| IBIS file stm32u375_385_wlcsp68-g_smps.ibs
[IBIS ver] 4.2
[File name] stm32u375_385_wlcsp68-g_smps.ibs
[File Rev] 1.2
[Date] 23-06-2025
[Source] Data Created at STMicroelectronics
[Notes]  File originated from ELDO simulations.
[Disclaimer]  This information is for modeling purpose only and is
   not guaranted. The information is subject to change without
   notice.
[Copyright] Copyright 2025 STMicroelectronics Inc.
|   Component stm32u375_385_wlcsp68-g_smps
[Component] stm32u375_385_wlcsp68-g_smps
[Manufacturer] STMicroelectronics
[Package]
| variable   typ   min   max
R_pkg  0  NA  NA
L_pkg  0  NA  NA
C_pkg  0  NA  NA
[Pin]   signal_name   model_name
A1  VDDUSB  power
A3  PG10  io8_ft_100m_hslv
A5  VDDIO2  power
A7  PB7  io8_ft_100m_hslv
A9  VDD  power
B2  VDD  power
B4  PG14  io8_ft_100m_hslv
B6  PB4  io8_ft_100m_hslv
B8  PH3-BOOT0  io8_ft_100m_hslv
C1  PA12  io8usb_ft_phy
C3  PG9  io8_ft_100m_hslv
C5  VSS  gnd
C7  PB6  io8_ft_100m_hslv
C9  VBAT  power
D2  VSS  gnd
D4  PG12  io8_ft_100m_hslv
D6  PB3  io8_ft_100m_hslv
D8  VSS  gnd
E1  PA11  io8usb_ft_phy
E3  PA15  io8_ft_100m
E5  PG13  io8_ft_100m_hslv
E7  PB5  io8_ft_100m_hslv
E9  PC14-OSC32_IN  io_ft_tamp
F2  PA10  io8_ft_100m
F4  PA14  io8_ft_100m
F6  PG15  io8_ft_100m_hslv
F8  PC13  io8_ft_100m_v33
G1  VDDIO2  power
G3  PA9  io8_ft_100m
G5  PG11  io8_ft_100m_hslv
G7  NRST  ioreset_v33
G9  PC15-OSC32_OUT  io_ft_tamp
H2  VSS  gnd
H4  PA13  io8_ft_100m
H6  PA8  io8_ft_100m_hslv
H8  PH1-OSC_OUT  io8_ft_100m
J1  PG6  io8_ft_100m_hslv
J3  PG7  io8_ft_100m_hslv
J5  PG8  io8_ft_100m_hslv
J7  PA0  io8_ft_100m
J9  PH0-OSC_IN  io8_ft_100m
K2  PG4  io8_ft_100m_hslv
K4  PG5  io8_ft_100m_hslv
K6  PA5  io8_ft_100m
K8  VSSA  nc
L1  PG2  io8_ft_100m_hslv
L3  PB15  io8_ft_100m
L5  PG3  io8_ft_100m_hslv
L7  PA1  io8_ft_100m_hslv
L9  VDDA  nc
M2  PB14  io8_ft_100m_hslv
M4  PB13  io8_ft_100m_hslv
M6  PA7  io8_ft_100m_hslv
M8  PA2  io8_ft_100m_hslv
N1  VSS  gnd
N3  VSSSMPS  nc
N5  PB0  io8_ft_100m_hslv
N7  PA4  io8_ft_100m_hslv
N9  PA3  io8_ft_100m_hslv
P2  VDD11  nc
P4  VLXSMPS  nc
P6  PB1  io8_ft_100m_hslv
P8  VSS  gnd
R1  VDD  power
R3  VDDSMPS  nc
R5  PB2  io8_ft_100m_hslv
R7  PA6  io8_ft_100m_hslv
R9  VDD  power
[Package Model]   454-wlcsp68-portg-250418
[Pin Mapping]   pulldown_ref   pullup_ref   | Comment
A1  nc  vddusb
A3  gndio  vddio2
A5  nc  vddio2
A7  gndio  vddio
A9  nc  vddio
B2  nc  vddio
B4  gndio  vddio2
B6  gndio  vddio
B8  gndio  vddio
C1  gndio  vddusb  | Depending on IO usage
| C1  gndio  vddio  | Depending on IO usage
C3  gndio  vddio2
C5  gndio  nc
C7  gndio  vddio
C9  nc  vsw
D2  gndio  nc
D4  gndio  vddio2
D6  gndio  vddio
D8  gndio  nc
E1  gndio  vddusb  | Depending on IO usage
| E1  gndio  vddio  | Depending on IO usage
E3  gndio  vddio
E5  gndio  vddio2
E7  gndio  vddio
E9  gndio  vsw
F2  gndio  vddio
F4  gndio  vddio
F6  gndio  vddio2
F8  gndio  vsw
G1  nc  vddio2
G3  gndio  vddio
G5  gndio  vddio2
G7  gndio  vddio
G9  gndio  vsw
H2  gndio  nc
H4  gndio  vddio
H6  gndio  vddio
H8  gndio  vddio
J1  gndio  vddio2
J3  gndio  vddio2
J5  gndio  vddio2
J7  gndio  vddio
J9  gndio  vddio
K2  gndio  vddio2
K4  gndio  vddio2
K6  gndio  vddio
K8  nc  nc
L1  gndio  vddio2
L3  gndio  vddio
L5  gndio  vddio2
L7  gndio  vddio
L9  nc  nc
M2  gndio  vddio
M4  gndio  vddio
M6  gndio  vddio
M8  gndio  vddio
N1  gndio  nc
N3  nc  nc
N5  gndio  vddio
N7  gndio  vddio
N9  gndio  vddio
P2  nc  nc
P4  nc  nc
P6  gndio  vddio
P8  gndio  nc
R1  nc  vddio
R3  nc  nc
R5  gndio  vddio
R7  gndio  vddio
R9  nc  vddio
|[Diff Pin]  inv_pin  vdiff  tdelay_typ  tdelay_min  tdelay_max
|C1  E1  NA  NA  NA  NA
[Model Selector] io8_ft_100m
io8_ft_100m_ls_1v2  "GPIO 100MHz - 5V tolerant - low speed - 1.2V range"
io8_ft_100m_ls_1v8  "GPIO 100MHz - 5V tolerant - low speed - 1.8V range"
io8_ft_100m_ls_3v3  "GPIO 100MHz - 5V tolerant - low speed - 3.3V range"
io8_ft_100m_ms_1v2  "GPIO 100MHz - 5V tolerant - med speed - 1.2V range"
io8_ft_100m_ms_1v8  "GPIO 100MHz - 5V tolerant - med speed - 1.8V range"
io8_ft_100m_ms_3v3  "GPIO 100MHz - 5V tolerant - med speed - 3.3V range"
io8_ft_100m_fs_1v2  "GPIO 100MHz - 5V tolerant - fast speed - 1.2V range"
io8_ft_100m_fs_1v8  "GPIO 100MHz - 5V tolerant - fast speed - 1.8V range"
io8_ft_100m_fs_3v3  "GPIO 100MHz - 5V tolerant - fast speed - 3.3V range"
io8_ft_100m_hs_1v2  "GPIO 100MHz - 5V tolerant - high speed - 1.2V range"
io8_ft_100m_hs_1v8  "GPIO 100MHz - 5V tolerant - high speed - 1.8V range"
io8_ft_100m_hs_3v3  "GPIO 100MHz - 5V tolerant - high speed - 3.3V range"
[Model Selector] io8_ft_100m_hslv
io8_ft_100m_ls_1v2  "GPIO 100MHz - 5V tolerant - low speed - 1.2V range"
io8_ft_100m_ls_1v8  "GPIO 100MHz - 5V tolerant - low speed - 1.8V range"
io8_ft_100m_ls_3v3  "GPIO 100MHz - 5V tolerant - low speed - 3.3V range"
io8_ft_100m_ms_1v2  "GPIO 100MHz - 5V tolerant - med speed - 1.2V range"
io8_ft_100m_ms_1v8  "GPIO 100MHz - 5V tolerant - med speed - 1.8V range"
io8_ft_100m_ms_3v3  "GPIO 100MHz - 5V tolerant - med speed - 3.3V range"
io8_ft_100m_fs_1v2  "GPIO 100MHz - 5V tolerant - fast speed - 1.2V range"
io8_ft_100m_fs_1v8  "GPIO 100MHz - 5V tolerant - fast speed - 1.8V range"
io8_ft_100m_fs_3v3  "GPIO 100MHz - 5V tolerant - fast speed - 3.3V range"
io8_ft_100m_hs_1v2  "GPIO 100MHz - 5V tolerant - high speed - 1.2V range"
io8_ft_100m_hs_1v8  "GPIO 100MHz - 5V tolerant - high speed - 1.8V range"
io8_ft_100m_hs_3v3  "GPIO 100MHz - 5V tolerant - high speed - 3.3V range"
io8_ft_100m_hslv_ls_1v2  "GPIO 100MHz low voltage optimization - 5V tolerant - low speed - 1.2V range"
io8_ft_100m_hslv_ls_1v8  "GPIO 100MHz low voltage optimization - 5V tolerant - low speed - 1.8V range"
io8_ft_100m_hslv_ls_2v5  "GPIO 100MHz low voltage optimization - 5V tolerant - low speed - 3.3V range"
io8_ft_100m_hslv_ms_1v2  "GPIO 100MHz low voltage optimization - 5V tolerant - med speed - 1.2V range"
io8_ft_100m_hslv_ms_1v8  "GPIO 100MHz low voltage optimization - 5V tolerant - med speed - 1.8V range"
io8_ft_100m_hslv_ms_2v5  "GPIO 100MHz low voltage optimization - 5V tolerant - med speed - 3.3V range"
io8_ft_100m_hslv_fs_1v2  "GPIO 100MHz low voltage optimization - 5V tolerant - fast speed - 1.2V range"
io8_ft_100m_hslv_fs_1v8  "GPIO 100MHz low voltage optimization - 5V tolerant - fast speed - 1.8V range"
io8_ft_100m_hslv_fs_2v5  "GPIO 100MHz low voltage optimization - 5V tolerant - fast speed - 3.3V range"
io8_ft_100m_hslv_hs_1v2  "GPIO 100MHz low voltage optimization - 5V tolerant - high speed - 1.2V range"
io8_ft_100m_hslv_hs_1v8  "GPIO 100MHz low voltage optimization - 5V tolerant - high speed - 1.8V range"
io8_ft_100m_hslv_hs_2v5  "GPIO 100MHz low voltage optimization - 5V tolerant - high speed - 3.3V range"
[Model Selector] io8_ft_100m_v33
io8_ft_100m_v33_ls_1v2  "GPIO_V33 100MHz - 5V tolerant - low speed - 1.2V range"
io8_ft_100m_v33_ls_1v8  "GPIO_V33 100MHz - 5V tolerant - low speed - 1.8V range"
io8_ft_100m_v33_ls_3v3  "GPIO_V33 100MHz - 5V tolerant - low speed - 3.3V range"
io8_ft_100m_v33_ms_1v2  "GPIO_V33 100MHz - 5V tolerant - med speed - 1.2V range"
io8_ft_100m_v33_ms_1v8  "GPIO_V33 100MHz - 5V tolerant - med speed - 1.8V range"
io8_ft_100m_v33_ms_3v3  "GPIO_V33 100MHz - 5V tolerant - med speed - 3.3V range"
io8_ft_100m_v33_fs_1v2  "GPIO_V33 100MHz - 5V tolerant - fast speed - 1.2V range"
io8_ft_100m_v33_fs_1v8  "GPIO_V33 100MHz - 5V tolerant - fast speed - 1.8V range"
io8_ft_100m_v33_fs_3v3  "GPIO_V33 100MHz - 5V tolerant - fast speed - 3.3V range"
io8_ft_100m_v33_hs_1v2  "GPIO_V33 100MHz - 5V tolerant - high speed - 1.2V range"
io8_ft_100m_v33_hs_1v8  "GPIO_V33 100MHz - 5V tolerant - high speed - 1.8V range"
io8_ft_100m_v33_hs_3v3  "GPIO_V33 100MHz - 5V tolerant - high speed - 3.3V range"
[Model Selector] io8usb_ft_phy
io8_ft_100m_ls_1v2  "GPIO 100MHz - 5V tolerant - low speed - 1.2V range"
io8_ft_100m_ls_1v8  "GPIO 100MHz - 5V tolerant - low speed - 1.8V range"
io8_ft_100m_ls_3v3  "GPIO 100MHz - 5V tolerant - low speed - 3.3V range"
io8_ft_100m_ms_1v2  "GPIO 100MHz - 5V tolerant - med speed - 1.2V range"
io8_ft_100m_ms_1v8  "GPIO 100MHz - 5V tolerant - med speed - 1.8V range"
io8_ft_100m_ms_3v3  "GPIO 100MHz - 5V tolerant - med speed - 3.3V range"
io8_ft_100m_fs_1v2  "GPIO 100MHz - 5V tolerant - fast speed - 1.2V range"
io8_ft_100m_fs_1v8  "GPIO 100MHz - 5V tolerant - fast speed - 1.8V range"
io8_ft_100m_fs_3v3  "GPIO 100MHz - 5V tolerant - fast speed - 3.3V range"
io8_ft_100m_hs_1v2  "GPIO 100MHz - 5V tolerant - high speed - 1.2V range"
io8_ft_100m_hs_1v8  "GPIO 100MHz - 5V tolerant - high speed - 1.8V range"
io8_ft_100m_hs_3v3  "GPIO 100MHz - 5V tolerant - high speed - 3.3V range"
io8usb_ft_phy_hs_3v3   "USB full speed"
io8usb_ft_phy_ls_3v3   "USB low speed"
[Model Selector] io_ft_tamp
io_ft_tamp_ls_1v2 "io8_ft tamp low speed @ 1.2V"
io_ft_tamp_ls_1v8 "io8_ft tamp low speed @ 1.8V"
io_ft_tamp_ls_3v3 "io8_ft tamp low speed @ 3.3V"
io_ft_tamp_ms_1v2 "io8_ft tamp med speed @ 1.2V"
io_ft_tamp_ms_1v8 "io8_ft tamp med speed @ 1.8V"
io_ft_tamp_ms_3v3 "io8_ft tamp med speed @ 3.3V"
io_ft_tamp_fs_1v2 "io8_ft tamp fast speed @ 1.2V"
io_ft_tamp_fs_1v8 "io8_ft tamp fast speed @ 1.8V"
io_ft_tamp_fs_3v3 "io8_ft tamp fast speed @ 3.3V"
io_ft_tamp_hs_1v2 "io8_ft tamp high speed @ 1.2V"
io_ft_tamp_hs_1v8 "io8_ft tamp high speed @ 1.8V"
io_ft_tamp_hs_3v3 "io8_ft tamp high speed @ 3.3V"
[Model Selector] ioreset_v33
ioreset_v33_1v2 "Reset PAD. 5V tolerant. 1.2V range"
ioreset_v33_1v8 "Reset PAD. 5V tolerant. 1.8V range"
ioreset_v33_3v3 "Reset PAD. 5V tolerant. 3.3V range"
[Define Package Model]  454-wlcsp68-portg-250418
[Manufacturer]  Unknown
[OEM]  Unknown
[Description]  None
[Number Of Pins]  65
[Pin Numbers]
| Pin Num   Terminal Name
G7 | NRST
J7 | PA0
L7 | PA1
M8 | PA2
N9 | PA3
N7 | PA4
K6 | PA5
R7 | PA6
M6 | PA7
H6 | PA8
G3 | PA9
F2 | PA10
E1 | PA11
C1 | PA12
H4 | PA13
F4 | PA14
E3 | PA15
N5 | PB0
P6 | PB1
R5 | PB2
D6 | PB3
B6 | PB4
E7 | PB5
C7 | PB6
A7 | PB7
M4 | PB13
M2 | PB14
L3 | PB15
F8 | PC13
E9 | PC14-OSC32_IN
G9 | PC15-OSC32_OUT
L1 | PG2
L5 | PG3
K2 | PG4
K4 | PG5
J1 | PG6
J3 | PG7
J5 | PG8
C3 | PG9
A3 | PG10
G5 | PG11
D4 | PG12
E5 | PG13
B4 | PG14
F6 | PG15
J9 | PH0-OSC_IN
H8 | PH1-OSC_OUT
B8 | PH3-BOOT0
P2 | VDD11
C9 | VBAT
A9 | VDD
B2 | VDD
R1 | VDD
R9 | VDD
L9 | VDDA
G1 | VDDIO2
A5 | VDDIO2
R3 | VDDSMPS
A1 | VDDUSB
P4 | VLXSMPS
C5 | VSS
D2 | VSS
H2 | VSS
K8 | VSSA
N3 | VSSSMPS
|[Merged Pins]  C5
|D8  |  VSS
|N1  |  VSS
|P8  |  VSS
[Model Data]
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[End Model Data]
[End Package Model]
|End [Component]
| Models and submodels in the file (53): io8_ft_100m_fs_1v2 (I/O), io8_ft_100m_fs_1v8 (I/O), io8_ft_100m_fs_3v3 (I/O), io8_ft_100m_hs_1v2 (I/O), io8_ft_100m_hs_1v8 (I/O), io8_ft_100m_hs_3v3 (I/O), io8_ft_100m_hslv_fs_1v2 (I/O), io8_ft_100m_hslv_fs_1v8 (I/O), io8_ft_100m_hslv_fs_2v5 (I/O), io8_ft_100m_hslv_hs_1v2 (I/O), io8_ft_100m_hslv_hs_1v8 (I/O), io8_ft_100m_hslv_hs_2v5 (I/O), io8_ft_100m_hslv_ls_1v2 (I/O), io8_ft_100m_hslv_ls_1v8 (I/O), io8_ft_100m_hslv_ls_2v5 (I/O), io8_ft_100m_hslv_ms_1v2 (I/O), io8_ft_100m_hslv_ms_1v8 (I/O), io8_ft_100m_hslv_ms_2v5 (I/O), io8_ft_100m_ls_1v2 (I/O), io8_ft_100m_ls_1v8 (I/O), io8_ft_100m_ls_3v3 (I/O), io8_ft_100m_ms_1v2 (I/O), io8_ft_100m_ms_1v8 (I/O), io8_ft_100m_ms_3v3 (I/O), io8_ft_100m_v33_fs_1v2 (I/O), io8_ft_100m_v33_fs_1v8 (I/O), io8_ft_100m_v33_fs_3v3 (I/O), io8_ft_100m_v33_hs_1v2 (I/O), io8_ft_100m_v33_hs_1v8 (I/O), io8_ft_100m_v33_hs_3v3 (I/O), io8_ft_100m_v33_ls_1v2 (I/O), io8_ft_100m_v33_ls_1v8 (I/O), io8_ft_100m_v33_ls_3v3 (I/O), io8_ft_100m_v33_ms_1v2 (I/O), io8_ft_100m_v33_ms_1v8 (I/O), io8_ft_100m_v33_ms_3v3 (I/O), io8usb_ft_phy_hs_3v3 (I/O), io8usb_ft_phy_ls_3v3 (I/O), io_ft_tamp_fs_1v2 (I/O), io_ft_tamp_fs_1v8 (I/O), io_ft_tamp_fs_3v3 (I/O), io_ft_tamp_hs_1v2 (I/O), io_ft_tamp_hs_1v8 (I/O), io_ft_tamp_hs_3v3 (I/O), io_ft_tamp_ls_1v2 (I/O), io_ft_tamp_ls_1v8 (I/O), io_ft_tamp_ls_3v3 (I/O), io_ft_tamp_ms_1v2 (I/O), io_ft_tamp_ms_1v8 (I/O), io_ft_tamp_ms_3v3 (I/O), ioreset_v33_1v2 (I/O_open_drain), ioreset_v33_1v8 (I/O_open_drain), ioreset_v33_3v3 (I/O_open_drain)
